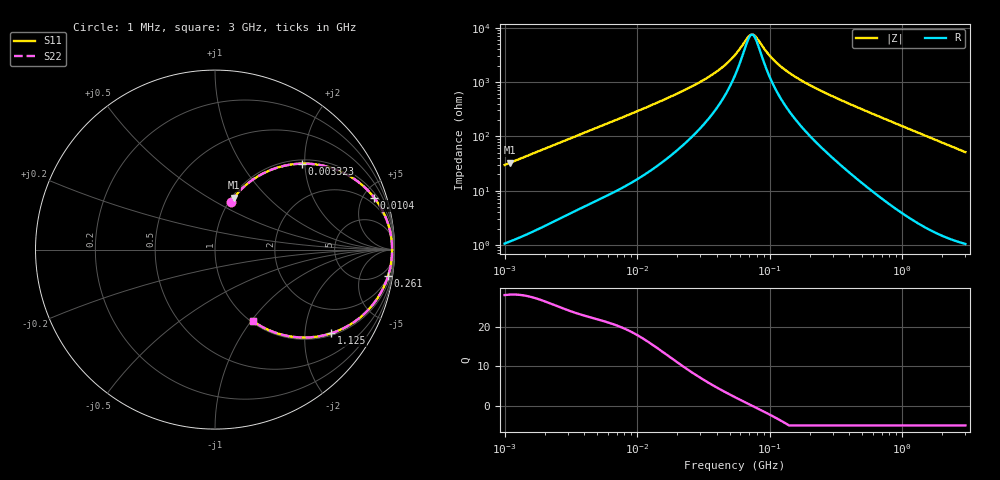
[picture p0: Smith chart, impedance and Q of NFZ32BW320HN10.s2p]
! NFZ32BW320HN10
# Hz S RI R 50
!Freq.(Hz) S11(Real) S11(Imag) S21(Real) S21(Imag) S12(Real) S12(Imag) S22(Real) S22(Imag)
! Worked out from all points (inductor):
!   401 points, 1 MHz to 3 GHz, reference 50 ohm
!   read as one part in series: L = 4.7 uH near 1.041 MHz
!   highest Q = 28.1 at 1.105 MHz (marker M1), where L = 4.72 uH
!   self-resonance near 72.49 MHz
!   S11 on the Smith chart (normalised r, x): 1 MHz: 1.02, +0.59; 3.323 MHz: 1.08, +1.93; 10.4 MHz: 1.34, +6.02; 261 MHz: 2, -13; 1.125 GHz: 1.06, -2.74; 3 GHz: 1.02, -1.02
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1000000  0.089 0.2675  0.911 -0.2675  0.911 -0.2675  0.089 0.2675
1105259  0.1053 0.2896  0.8947 -0.2896  0.8947 -0.2896  0.1053 0.2896
1859846  0.2384 0.4079  0.7616 -0.4079  0.7616 -0.4079  0.2384 0.4079
3323290  0.4836 0.479  0.5164 -0.479  0.5164 -0.479  0.4836 0.479
3823119  0.5493 0.4763  0.4507 -0.4763  0.4507 -0.4763  0.5493 0.4763
6433254  0.7639 0.4013  0.2361 -0.4013  0.2361 -0.4013  0.7639 0.4013
1.040059e7  0.8876 0.2887  0.1124 -0.2887  0.1124 -0.2887  0.8876 0.2887
1.461624e7  0.9354 0.2133  0.0646 -0.2133  0.0646 -0.2133  0.9354 0.2133
3.387922e7  0.98 0.0795  0.02 -0.0795  0.02 -0.0795  0.98 0.0795
4.483659e7  0.9843 0.0482  0.0157 -0.0482  0.0157 -0.0482  0.9843 0.0482
5.477226e7  0.986 0.0281  0.014 -0.0281  0.014 -0.0281  0.986 0.0281
6.826239e7  0.9868 0.00711  0.0132 -0.00711  0.0132 -0.00711  0.9868 0.00711
7.544761e7  0.9869 -0.00226  0.0131 0.00226  0.0131 0.00226  0.9869 -0.00226
9.984923e7  0.9861 -0.0289  0.0139 0.0289  0.0139 0.0289  0.9861 -0.0289
1.171891e8  0.9849 -0.0449  0.0151 0.0449  0.0151 0.0449  0.9849 -0.0449
2.094008e8  0.9733 -0.1149  0.0267 0.1149  0.0267 0.1149  0.9733 -0.1149
2.609752e8  0.9638 -0.1489  0.0362 0.1489  0.0362 0.1489  0.9638 -0.1489
4.853736e8  0.9024 -0.2752  0.0976 0.2752  0.0976 0.2752  0.9024 -0.2752
8.005644e8  0.7819 -0.3987  0.2181 0.3987  0.2181 0.3987  0.7819 -0.3987
1.125055e9  0.6487 -0.4659  0.3513 0.4659  0.3513 0.4659  0.6487 -0.4659
1.782824e9  0.4275 -0.4851  0.5725 0.4851  0.5725 0.4851  0.4275 -0.4851
3e9  0.2122 -0.3988  0.7878 0.3988  0.7878 0.3988  0.2122 -0.3988
